PROGRAM PRG_DatFileCreat
VAR
	iSeq 			: INT;
	iExceptionSeq	: INT;	
	fbGetSystemTime	: NT_GetTime;
	
	i 				: INT;
	
	DatHeader		: stDatHeader;		(* Beware memory alignment *)
	DatAcqBlock		: stAcquisitionBlock;
	pRequestData	: POINTER TO BOOL;
	
	nCurRecodeNo	: UDINT;	
	
	sFileName		: T_MaxString;
	
	
	fbFileOpen		: FB_FileOpen;
	fbFileSeek		: FB_FileSeek;
	fbFileWrite		: FB_FileWrite;
	fbFileClose		: FB_FileClose;
	
	nTxtParserLate	: UDINT;		(* Lag counter *)
	pPathPassThrough	: 	POINTER TO T_MaxString;
	pStartParser	: POINTER TO BOOL;
	
END_VAR

pRequestData := ADR(MAIN.fbBufferAccess.bGetData);

CASE iSeq OF
0:	(* Check for bSamplingStart command start *)
	IF NOT(MAIN.fbBufferAccess.bFifoEmpty) THEN
		nCurRecodeNo := 0;
		iSeq := iSeq + 1;
	END_IF
1:	(* Creat time serial file name *)
	fbGetSystemTime(NETID:= , 
		START:= TRUE, 
		TMOUT:= DEFAULT_ADS_TIMEOUT, 
		BUSY=> , 
		ERR=> , 
		ERRID=> , 
		TIMESTR=> );
	
	IF 	NOT(fbGetSystemTime.BUSY) AND NOT(fbGetSystemTime.ERR) THEN
(*
		iTemp := iTemp + 1;
		sFileName := USINT_TO_STRING(iTemp);
		sFileName := CONCAT (sFileName,'.dat');	
*)

		sFileName := SYSTEMTIME_TO_STRING(fbGetSystemTime.TIMESTR);

		fbGetSystemTime(START:= FALSE); 
		iSeq := iSeq + 1;
	ELSIF fbGetSystemTime.ERR THEN			
		fbGetSystemTime(START:= FALSE); 
		iExceptionSeq := iSeq;
		iSeq := 999;
	END_IF
2:	(*  fliter file name & creat further info  *)
	FOR i := 1 TO len(sFileName) BY 1 DO
		IF  F_ReplaceByString(sSource:= sFileName, sFindContent:= ':', sReplaceContent:='_' ) <> '' THEN	(* Replace content to avoid involid file name *)
			sFileName := F_ReplaceByString(sSource:= sFileName, sFindContent:= ':', sReplaceContent:='_' );
		ELSE
			EXIT;
		END_IF
	END_FOR			
		
	sFileName := CONCAT (sFileName,'Node_');
	sFileName := CONCAT (sFileName,INT_TO_STRING(MAIN.nAcuNodeId));
	sFileName := CONCAT (sFileName,'.dat');		(* add bin file extension *)
	iSeq := iSeq + 1;
3:	(* Creat file *)
	fbFileOpen.sPathName := CONCAT (sAccessPath, sFileName);

	fbFileOpen(sNetId:= sFileTargetNetId,			(* Access target id  *)
		sPathName:= ,	(* Access Path *)
		nMode:= FOPEN_MODEBINARY OR FOPEN_MODEWRITE,		(* Binary Format & Write Mode & Overrite contents   *)
		ePath:= PATH_GENERIC,
		bExecute:= TRUE,
		tTimeout:= DEFAULT_ADS_TIMEOUT,
		bBusy=> ,
		bError=> ,
		nErrId=> ,
		hFile=> );
		
	IF 	NOT(fbFileOpen.bBusy) AND NOT(fbFileOpen.bError) THEN
		fbFileOpen(bExecute:= FALSE);
		iSeq := iSeq + 1;
	ELSIF fbFileOpen.bError THEN
		fbFileOpen(bExecute:= FALSE);
		iExceptionSeq := iSeq;
		iSeq := 999;
	END_IF
		
4:	(* Creat binary info header *)
	fbFileWrite(sNetId:= sFileTargetNetId, 
		hFile:= fbFileOpen.hFile, 
		pWriteBuff:= ADR(DatHeader), 
		cbWriteLen:= SIZEOF(DatHeader), 
		bExecute:= TRUE, 
		tTimeout:= DEFAULT_ADS_TIMEOUT, 
		bBusy=> , 
		bError=> , 
		nErrId=> , 
		cbWrite=> );

	IF NOT(fbFileWrite.bBusy) AND NOT(fbFileWrite.bError) THEN
		fbFileWrite(bExecute:= FALSE);
		iSeq := iSeq + 1;
	ELSIF fbFileWrite.bError THEN
		fbFileWrite(bExecute:= FALSE);
		iExceptionSeq := iSeq;
		iSeq := 999;
	END_IF
5:	(* seek to cyclic record position  *)
	fbFileSeek(sNetId:= sFileTargetNetId, 
		hFile:= fbFileOpen.hFile, 
		nSeekPos:= SIZEOF(DatHeader), 		(* Seek to record start position *)
		eOrigin:= SEEK_SET, 
		bExecute:= , 
		tTimeout:= DEFAULT_ADS_TIMEOUT, 
		bBusy=> , 
		bError=> , 
		nErrId=> );
		
	IF NOT(fbFileSeek.bBusy) AND NOT(fbFileSeek.bError) THEN
		fbFileSeek(bExecute:= FALSE);
		iSeq := 10;
	ELSIF fbFileSeek.bError THEN
		fbFileSeek(bExecute:= FALSE);
		iExceptionSeq := iSeq;
		iSeq := 999;
	END_IF

10:		(* Check Data exist *)
	IF NOT(MAIN.fbBufferAccess.bFifoEmpty) THEN		
		pRequestData^ := TRUE;			(* request get data from buffer to DatAcqBlock *)
		iSeq := iSeq + 1;
	END_IF
11:
	fbFileWrite(sNetId:= sFileTargetNetId, 
		hFile:= fbFileOpen.hFile, 
		pWriteBuff:= ADR(DatAcqBlock), 
		cbWriteLen:= SIZEOF(DatAcqBlock), 
		bExecute:= TRUE, 
		tTimeout:= DEFAULT_ADS_TIMEOUT, 
		bBusy=> , 
		bError=> , 
		nErrId=> , 
		cbWrite=> );

	IF NOT(fbFileWrite.bBusy) AND NOT(fbFileWrite.bError) THEN
		fbFileWrite(bExecute:= FALSE);
		iSeq := iSeq + 1;
	ELSIF fbFileWrite.bError THEN
		fbFileWrite(bExecute:= FALSE);
		iExceptionSeq := iSeq;
		iSeq := 999;
	END_IF
12:	(* Seek to next block *)
	fbFileSeek(sNetId:= sFileTargetNetId, 
		hFile:= fbFileOpen.hFile, 
		nSeekPos:= fbFileSeek.nSeekPos + SIZEOF(DatAcqBlock), 		(* Seek to record start position *)
		eOrigin:= SEEK_SET, 
		bExecute:= , 
		tTimeout:= DEFAULT_ADS_TIMEOUT, 
		bBusy=> , 
		bError=> , 
		nErrId=> );
		
	IF NOT(fbFileSeek.bBusy) AND NOT(fbFileSeek.bError) THEN
		fbFileSeek(bExecute:= FALSE);
		iSeq := iSeq + 1;
	ELSIF fbFileSeek.bError THEN
		fbFileSeek(bExecute:= FALSE);
		iExceptionSeq := iSeq;
		iSeq := 999;
	END_IF
13:	(*  Check if the record times & length reached  *)
	nCurRecodeNo := nCurRecodeNo + 1;
	IF nCurRecodeNo >= nRecordAcqBlockPerFile THEN
		iSeq := 20;		(* FileClose & creat New file *)
	ELSE
		iSeq := 10;		(* GobBack do further content write *)
	END_IF

	
20:	(* File Close *)
	fbFileClose(sNetId:= sFileTargetNetId, 
		hFile:= fbFileOpen.hFile,  
		bExecute:= TRUE, 
		tTimeout:= DEFAULT_ADS_TIMEOUT, 
		bBusy=> , 
		bError=> , 
		nErrId=> );

	IF NOT(fbFileClose.bBusy) AND NOT(fbFileClose.bError) THEN
		fbFileClose(bExecute:= FALSE);
		iSeq := iSeq + 1;
	ELSIF fbFileSeek.bError THEN
		fbFileClose(bExecute:= FALSE);
		iExceptionSeq := iSeq;
		iSeq := 999;
	END_IF
21:	(* Option call bin to txt file parser process *)
	pStartParser := ADR (PRG_Slow.fbTxtParser.bExecute);
	IF PRG_Slow.fbTxtParser.bBusy THEN			(* Parser process to slower then cyclic acquisition *)
		nTxtParserLate := nTxtParserLate + 1;
	ELSE
		pPathPassThrough := ADR(PRG_Slow.fbTxtParser.sFilePathSource); 
		pPathPassThrough^ := fbFileOpen.sPathName;

		pPathPassThrough := ADR(PRG_Slow.fbTxtParser.sFilePathDestination);
		pPathPassThrough^ := F_ReplaceByString(fbFileOpen.sPathName,'.dat' , '.csv');
	
		pStartParser^ := TRUE;
		iSeq := 0;
	END_IF
END_CASE

END_PROGRAM
